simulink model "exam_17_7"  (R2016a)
settings: Solver=ode23tb  StartTime=0.0  StopTime=0.2  RelTol=1e-3
libraries: powerlib x11

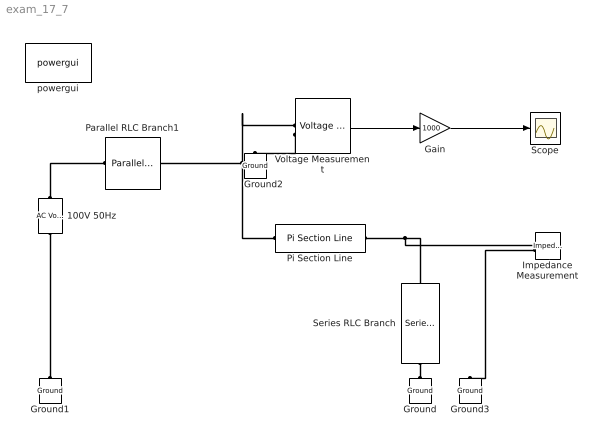
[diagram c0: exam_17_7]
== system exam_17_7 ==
  100V 50Hz : powerlib/Electrical Sources/AC Voltage Source  Amplitude=100  Phase=0  Frequency=50  SampleTime=0  Measurements=None  BusType=swing  Pref=10e3  Qref=0  Qmin=-inf  Qmax=+inf
  Gain : Gain  Gain=1000
  Ground{,1..3} (4 alike) : powerlib/Elements/Ground  LConnTagsString=a
  Impedance Measurement : powerlib/Measurements/Impedance Measurement  LConnTagsString=+|-  Factor=1
  Parallel RLC Branch1 : powerlib/Elements/Parallel RLC Branch  LConnTagsString=a  RConnTagsString=__new0  BranchType=R  Resistance=1  Inductance=1e-3  SetiL0=off  InitialCurrent=0  Capacitance=1e-6  Setx0=off  InitialVoltage=0  Measurements=None
  Pi Section Line : powerlib/Elements/Pi Section Line  LConnTagsString=__new0  RConnTagsString=__new0  Frequency=50  Resistance=0.1  Inductance=1.6e-3  Capacitance=10.2e-9  Length=300  PiSections=1  Measurements=None
  Scope : Scope
  Series RLC Branch : powerlib/Elements/Series RLC Branch  LConnTagsString=__new0  RConnTagsString=__new0  BranchType=RL  Resistance=1  Inductance=1  SetiL0=off  InitialCurrent=0  Capacitance=3.06  Setx0=off  InitialVoltage=0  Measurements=None
  Voltage Measurement : powerlib/Measurements/Voltage Measurement  PhasorSimulation=off  OutputType=Complex  PSBequivalent=0
  powergui : powerlib/powergui  Priority=1  SimulationMode=Continuous  SolverType=Tustin/Backward Euler (TBE)  SampleTime=50e-6  frequency=60  SPID=off  DisableSnubberDevices=off  DisableRonSwitches=off  DisableVfSwitches=off  SwTol=0  DisplayEquations=off  Interpol=off  ExternalGateDelay=off  methode=off  Ts=10  FunctionMessages=off  echomessages=off  HookPort=off  EnableUseOfTLC=off  x0status=blocks  frequencyindice=50  Pbase=100e6  ErrMax=1e-4  Iterations=50  UnitsV=kV  UnitsW=MW  buscounter=0  RestoreLinks=warning  ResistiveCurrentMeasurement=off  Frange=[0:2:500]  Ylog=on  Xlog=off  ShowGrid=on  save=off  variable=ZData  structure=0  ZoomFFT=off  StartTime=0.0  cycles=1  DisplayStyle=1  fundamental=60  FreqAxis=off  MaxFrequency=1000  frequencyindicesteady=1  RmsSteady=1  display=off
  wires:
  Voltage Measurement/1 -> Gain/1
  Gain/1 -> Scope/1
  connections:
  Pi Section Line/RConn1 -- Impedance Measurement/LConn1 -- Series RLC Branch/LConn1
  Impedance Measurement/LConn2 -- Ground3/LConn1
  Pi Section Line/LConn1 -- Parallel RLC Branch1/RConn1 -- Voltage Measurement/LConn1
  Voltage Measurement/LConn2 -- Ground2/LConn1
  Ground/LConn1 -- Series RLC Branch/RConn1
  100V 50Hz/LConn1 -- Ground1/LConn1
  100V 50Hz/RConn1 -- Parallel RLC Branch1/LConn1
